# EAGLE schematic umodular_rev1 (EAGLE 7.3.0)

## Sheet 1 of 8: vco1
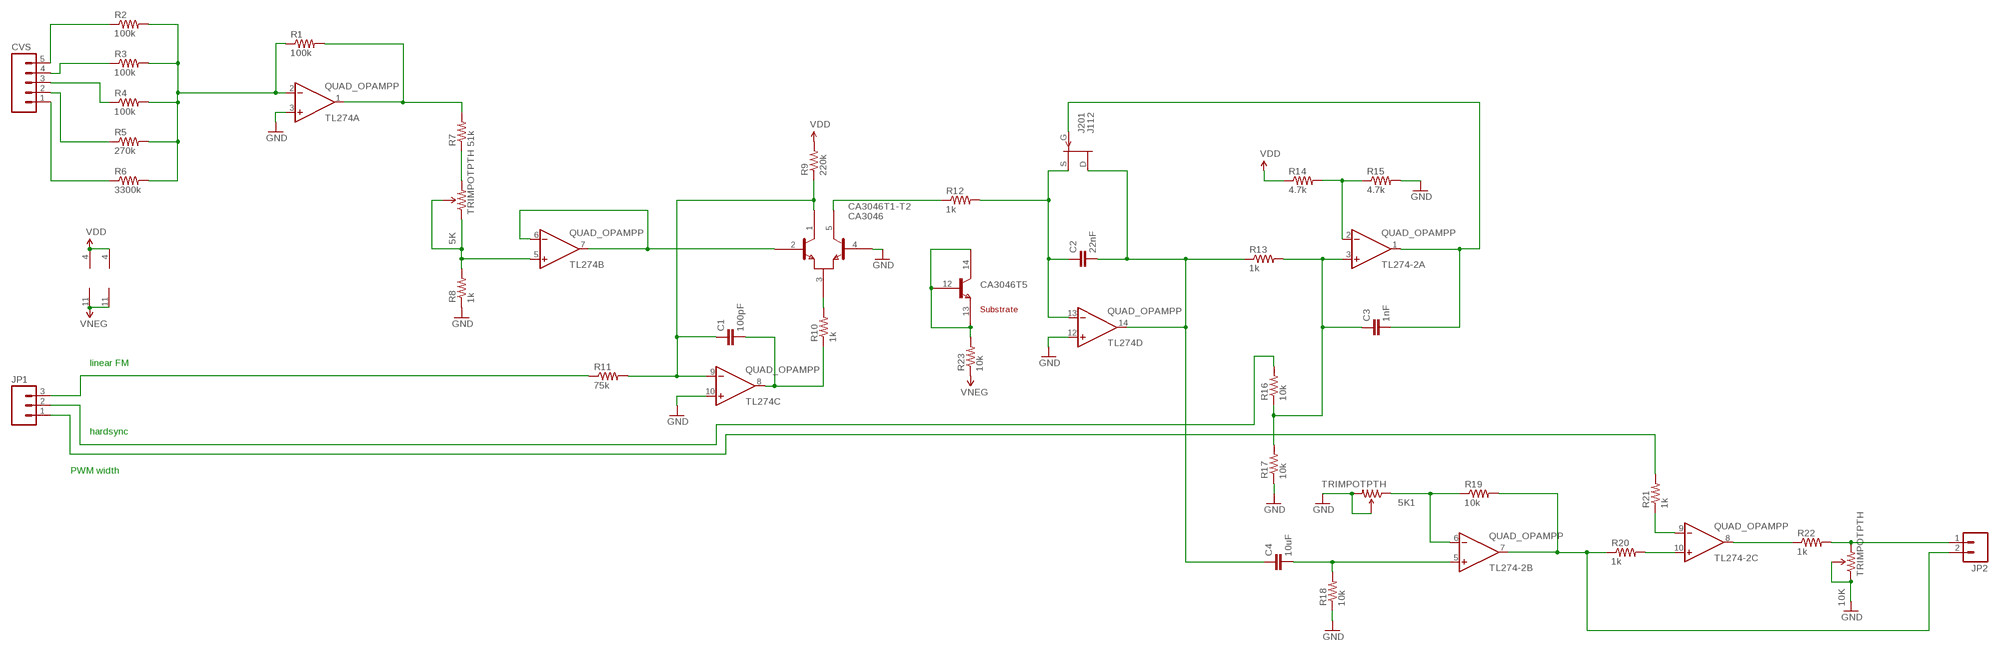
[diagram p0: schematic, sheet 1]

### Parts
5K  TRIMPOTPTH  [TRIM_POT_PTH]
5K1  TRIMPOTPTH  [TRIM_POT_PTH]
10K  TRIMPOTPTH  [TRIM_POT_PTH]
C1  100pF  CAPPTH  [CAP-PTH-SMALL]
C2  22nF  CAPPTH1  [CAP-PTH-5MM]
C3  1nF  CAPPTH  [CAP-PTH-SMALL]
C4  10uF  CAPPTH  [CAP-PTH-SMALL]
CA3046  CA3046  [DIL14]
CVS  M05LOCK_LONGPADS  [1X05_LOCK_LONGPADS]
J112  J201  [TO92]
JP1  M03LOCK_LONGPADS  [1X03_LOCK_LONGPADS]
JP2  M02LOCK_LONGPADS  [1X02_LOCK_LONGPADS]
R1  100k  RESISTORPTH-1/4W  [AXIAL-0.4]
R2  100k  RESISTORPTH-1/4W  [AXIAL-0.4]
R3  100k  RESISTORPTH-1/4W  [AXIAL-0.4]
R4  100k  RESISTORPTH-1/4W  [AXIAL-0.4]
R5  270k  RESISTORPTH-1/4W  [AXIAL-0.4]
R6  3300k  RESISTORPTH-1/4W  [AXIAL-0.4]
R7  51k  RESISTORPTH-1/4W  [AXIAL-0.4]
R8  1k  RESISTORPTH-1/4W  [AXIAL-0.4]
R9  220k  RESISTORPTH-1/4W  [AXIAL-0.4]
R10  1k  RESISTORPTH-1/4W  [AXIAL-0.4]
R11  75k  RESISTORPTH-1/4W  [AXIAL-0.4]
R12  1k  RESISTORPTH-1/4W  [AXIAL-0.4]
R13  1k  RESISTORPTH-1/4W  [AXIAL-0.4]
R14  4.7k  RESISTORPTH-1/4W  [AXIAL-0.4]
R15  4.7k  RESISTORPTH-1/4W  [AXIAL-0.4]
R16  10k  RESISTORPTH-1/4W  [AXIAL-0.4]
R17  10k  RESISTORPTH-1/4W  [AXIAL-0.4]
R18  10k  RESISTORPTH-1/4W  [AXIAL-0.4]
R19  10k  RESISTORPTH-1/4W  [AXIAL-0.4]
R20  1k  RESISTORPTH-1/4W  [AXIAL-0.4]
R21  1k  RESISTORPTH-1/4W  [AXIAL-0.4]
R22  1k  RESISTORPTH-1/4W  [AXIAL-0.4]
R23  10k  RESISTORPTH-1/4W  [AXIAL-0.4]
TL274  QUAD_OPAMPP  [DIL14]
TL274-2  QUAD_OPAMPP  [DIL14]

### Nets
GND: 5K1.2(WIPER) 5K1.3(CW) 10K.1(CCW) 10K.2(WIPER) CA3046.4(T1-T2:B2) R8.P$1 R15.P$2 R17.P$1 R18.P$1 TL274.3(A:+IN) TL274.10(C:+IN) TL274.12(D:+IN) ; also sheet 2,3,4,5,6,7,8
N$1: R1.P$1 R2.P$2 R3.P$2 R4.P$2 R5.P$2 R6.P$2 TL274.2(A:-IN)
N$2: R1.P$2 R7.P$2 TL274.1(A:OUT)
N$3: CVS.5 R2.P$1
N$4: CVS.4 R3.P$1
N$5: CVS.3 R4.P$1
N$6: CVS.2 R5.P$1
N$7: CVS.1 R6.P$1
N$8: 5K.3(CW) R7.P$1
N$9: 5K.1(CCW) 5K.2(WIPER) R8.P$2 TL274.5(B:+IN)
N$10: CA3046.2(T1-T2:B1) TL274.6(B:-IN) TL274.7(B:OUT)
N$11: JP1.3 R11.P$1
N$12: C1.2 R10.P$1 TL274.8(C:OUT)
N$13: CA3046.5(T1-T2:C2) R12.P$1
N$14: C1.1 CA3046.1(T1-T2:C1) R9.P$1 R11.P$2 TL274.9(C:-IN)
N$15: CA3046.3(T1-T2:E) R10.P$2
N$16: C2.1 J112.2(S) R12.P$2 TL274.13(D:-IN)
N$17: C2.2 C4.1 J112.3(D) R13.P$1 TL274.14(D:OUT)
N$18: R20.P$2 TL274-2.10(C:+IN)
N$19: C3.2 J112.1(G) TL274-2.1(A:OUT)
N$20: R21.P$1 TL274-2.9(C:-IN)
N$21: R14.P$2 R15.P$1 TL274-2.2(A:-IN)
N$22: JP1.1 R21.P$2
N$23: C3.1 R13.P$2 R16.P$1 R17.P$2 TL274-2.3(A:+IN)
N$24: JP1.2 R16.P$2
N$25: C4.2 R18.P$2 TL274-2.5(B:+IN)
N$26: 5K1.1(CCW) R19.P$1 TL274-2.6(B:-IN)
N$27: JP2.2 R19.P$2 R20.P$1 TL274-2.7(B:OUT)
N$28: R22.P$1 TL274-2.8(C:OUT)
N$29: 10K.3(CW) JP2.1 R22.P$2
N$31: CA3046.12(T5:B) CA3046.13(T5:E) CA3046.14(T5:C) R23.P$2
VDD: R9.P$2 R14.P$1 TL274-2.4(P:V+) TL274.4(P:V+) ; also sheet 2,3,4,5,6,7,8
VNEG: R23.P$1 TL274-2.11(P:V-) TL274.11(P:V-) ; also sheet 2,3,4,5,6,7,8
Unconnected: CA3046.6(T3:B) CA3046.7(T3:E) CA3046.8(T3:C) CA3046.9(T4:B) CA3046.10(T4:E) CA3046.11(T4:C) TL274-2.12(D:+IN) TL274-2.13(D:-IN) TL274-2.14(D:OUT)

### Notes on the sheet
- linear FM
- hardsync
- PWM width

## Sheet 2 of 8: vco2
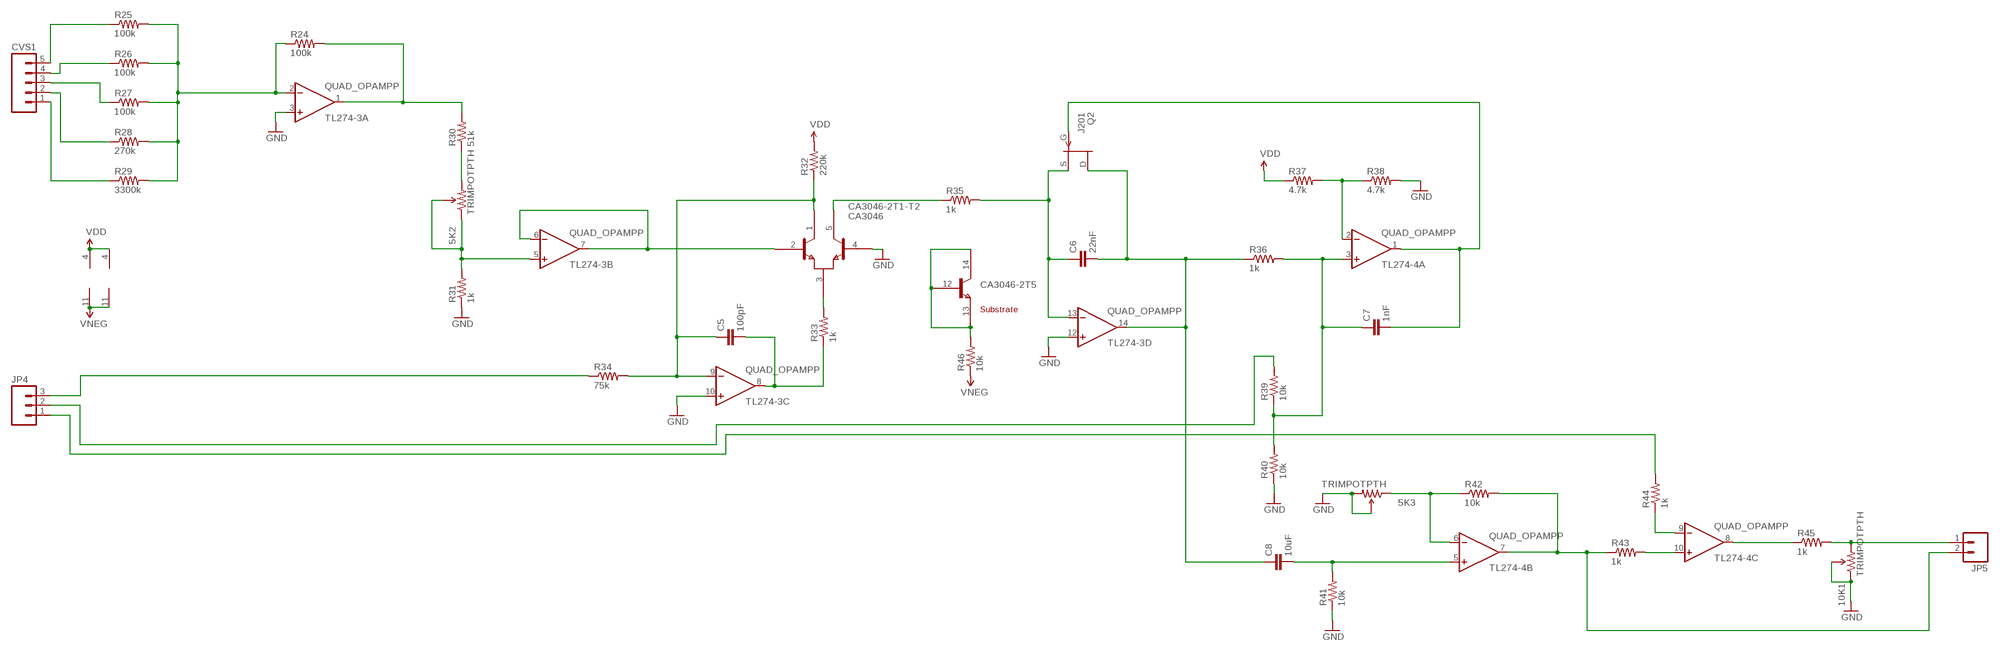
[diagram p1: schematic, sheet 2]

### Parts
5K2  TRIMPOTPTH  [TRIM_POT_PTH]
5K3  TRIMPOTPTH  [TRIM_POT_PTH]
10K1  TRIMPOTPTH  [TRIM_POT_PTH]
C5  100pF  CAPPTH  [CAP-PTH-SMALL]
C6  22nF  CAPPTH1  [CAP-PTH-5MM]
C7  1nF  CAPPTH  [CAP-PTH-SMALL]
C8  10uF  CAPPTH  [CAP-PTH-SMALL]
CA3046-2  CA3046  [DIL14]
CVS1  M05LOCK_LONGPADS  [1X05_LOCK_LONGPADS]
JP4  M03LOCK_LONGPADS  [1X03_LOCK_LONGPADS]
JP5  M02LOCK_LONGPADS  [1X02_LOCK_LONGPADS]
Q2  J201  [TO92]
R24  100k  RESISTORPTH-1/4W  [AXIAL-0.4]
R25  100k  RESISTORPTH-1/4W  [AXIAL-0.4]
R26  100k  RESISTORPTH-1/4W  [AXIAL-0.4]
R27  100k  RESISTORPTH-1/4W  [AXIAL-0.4]
R28  270k  RESISTORPTH-1/4W  [AXIAL-0.4]
R29  3300k  RESISTORPTH-1/4W  [AXIAL-0.4]
R30  51k  RESISTORPTH-1/4W  [AXIAL-0.4]
R31  1k  RESISTORPTH-1/4W  [AXIAL-0.4]
R32  220k  RESISTORPTH-1/4W  [AXIAL-0.4]
R33  1k  RESISTORPTH-1/4W  [AXIAL-0.4]
R34  75k  RESISTORPTH-1/4W  [AXIAL-0.4]
R35  1k  RESISTORPTH-1/4W  [AXIAL-0.4]
R36  1k  RESISTORPTH-1/4W  [AXIAL-0.4]
R37  4.7k  RESISTORPTH-1/4W  [AXIAL-0.4]
R38  4.7k  RESISTORPTH-1/4W  [AXIAL-0.4]
R39  10k  RESISTORPTH-1/4W  [AXIAL-0.4]
R40  10k  RESISTORPTH-1/4W  [AXIAL-0.4]
R41  10k  RESISTORPTH-1/4W  [AXIAL-0.4]
R42  10k  RESISTORPTH-1/4W  [AXIAL-0.4]
R43  1k  RESISTORPTH-1/4W  [AXIAL-0.4]
R44  1k  RESISTORPTH-1/4W  [AXIAL-0.4]
R45  1k  RESISTORPTH-1/4W  [AXIAL-0.4]
R46  10k  RESISTORPTH-1/4W  [AXIAL-0.4]
TL274-3  QUAD_OPAMPP  [DIL14]
TL274-4  QUAD_OPAMPP  [DIL14]

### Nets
GND: 5K3.2(WIPER) 5K3.3(CW) 10K1.1(CCW) 10K1.2(WIPER) CA3046-2.4(T1-T2:B2) R31.P$1 R38.P$2 R40.P$1 R41.P$1 TL274-3.3(A:+IN) TL274-3.10(C:+IN) TL274-3.12(D:+IN) ; also sheet 1,3,4,5,6,7,8
N$30: R24.P$1 R25.P$2 R26.P$2 R27.P$2 R28.P$2 R29.P$2 TL274-3.2(A:-IN)
N$32: R24.P$2 R30.P$2 TL274-3.1(A:OUT)
N$33: CVS1.5 R25.P$1
N$34: CVS1.4 R26.P$1
N$35: CVS1.3 R27.P$1
N$36: CVS1.2 R28.P$1
N$37: CVS1.1 R29.P$1
N$38: 5K2.3(CW) R30.P$1
N$39: 5K2.1(CCW) 5K2.2(WIPER) R31.P$2 TL274-3.5(B:+IN)
N$40: CA3046-2.2(T1-T2:B1) TL274-3.6(B:-IN) TL274-3.7(B:OUT)
N$41: C5.2 R33.P$1 TL274-3.8(C:OUT)
N$42: C5.1 CA3046-2.1(T1-T2:C1) R32.P$1 R34.P$2 TL274-3.9(C:-IN)
N$43: CA3046-2.3(T1-T2:E) R33.P$2
N$44: JP4.3 R34.P$1
N$45: CA3046-2.5(T1-T2:C2) R35.P$1
N$46: C6.1 Q2.2(S) R35.P$2 TL274-3.13(D:-IN)
N$47: C6.2 C8.1 Q2.3(D) R36.P$1 TL274-3.14(D:OUT)
N$48: C7.2 Q2.1(G) TL274-4.1(A:OUT)
N$49: R37.P$2 R38.P$1 TL274-4.2(A:-IN)
N$50: C7.1 R36.P$2 R39.P$1 R40.P$2 TL274-4.3(A:+IN)
N$51: JP4.2 R39.P$2
N$52: C8.2 R41.P$2 TL274-4.5(B:+IN)
N$53: 5K3.1(CCW) R42.P$1 TL274-4.6(B:-IN)
N$54: JP5.2 R42.P$2 R43.P$1 TL274-4.7(B:OUT)
N$55: R43.P$2 TL274-4.10(C:+IN)
N$56: R44.P$1 TL274-4.9(C:-IN)
N$57: JP4.1 R44.P$2
N$58: R45.P$1 TL274-4.8(C:OUT)
N$59: 10K1.3(CW) JP5.1 R45.P$2
N$60: CA3046-2.12(T5:B) CA3046-2.13(T5:E) CA3046-2.14(T5:C) R46.P$2
VDD: R32.P$2 R37.P$1 TL274-3.4(P:V+) TL274-4.4(P:V+) ; also sheet 1,3,4,5,6,7,8
VNEG: R46.P$1 TL274-3.11(P:V-) TL274-4.11(P:V-) ; also sheet 1,3,4,5,6,7,8
Unconnected: CA3046-2.6(T3:B) CA3046-2.7(T3:E) CA3046-2.8(T3:C) CA3046-2.9(T4:B) CA3046-2.10(T4:E) CA3046-2.11(T4:C) TL274-4.12(D:+IN) TL274-4.13(D:-IN) TL274-4.14(D:OUT)

## Sheet 3 of 8: pwr
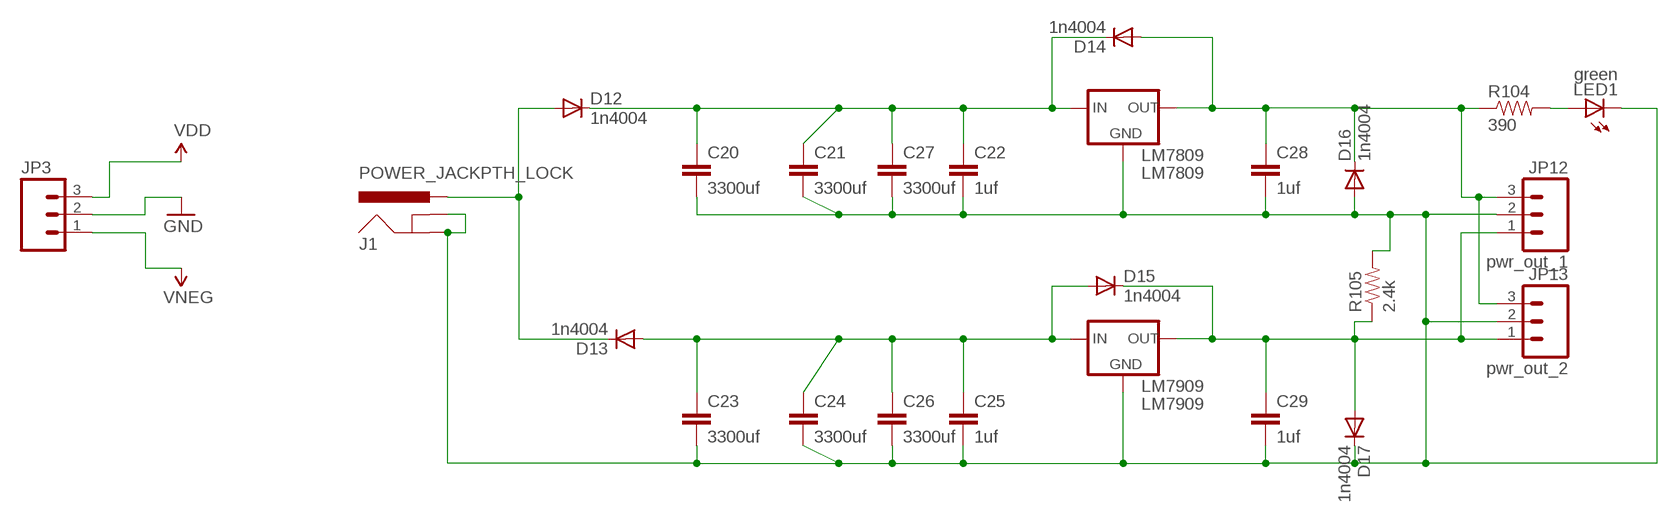
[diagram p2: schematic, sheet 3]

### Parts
C20  3300uf  CAPPTH3  [CAP-PTH-LARGE]
C21  3300uf  CAPPTH3  [CAP-PTH-LARGE]
C22  1uf  CAPPTH1  [CAP-PTH-5MM]
C23  3300uf  CAPPTH3  [CAP-PTH-LARGE]
C24  3300uf  CAPPTH3  [CAP-PTH-LARGE]
C25  1uf  CAPPTH1  [CAP-PTH-5MM]
C26  3300uf  CAPPTH3  [CAP-PTH-LARGE]
C27  3300uf  CAPPTH3  [CAP-PTH-LARGE]
C28  1uf  CAPPTH1  [CAP-PTH-5MM]
C29  1uf  CAPPTH1  [CAP-PTH-5MM]
D12  1n4004  DIODEPTH  [DIODE-1N4001]
D13  1n4004  DIODEPTH  [DIODE-1N4001]
D14  1n4004  DIODEPTH  [DIODE-1N4001]
D15  1n4004  DIODEPTH  [DIODE-1N4001]
D16  1n4004  DIODEPTH  [DIODE-1N4001]
D17  1n4004  DIODEPTH  [DIODE-1N4001]
J1  POWER_JACKPTH_LOCK  [POWER_JACK_PTH_LOCK]
JP3  M03LOCK_LONGPADS  [1X03_LOCK_LONGPADS]
JP12  pwr_out_1  M03LOCK_LONGPADS  [1X03_LOCK_LONGPADS]
JP13  pwr_out_2  M03LOCK_LONGPADS  [1X03_LOCK_LONGPADS]
LED1  green  LED3MM  [LED3MM]
LM7809  LM7809  V_REG_78XX-TO-220  [TO-220-ALT]
LM7909  LM7909  V_REG_78XX-TO-220  [TO-220-ALT]
R104  390  RESISTORPTH-1/4W  [AXIAL-0.4]
R105  2.4k  RESISTORPTH-1/4W  [AXIAL-0.4]

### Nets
GND: JP3.2 ; also sheet 1,2,4,5,6,7,8
N$150: D12.A D13.C J1.PWR
N$151: C20.1 C21.1 C22.1 C27.1 D12.C D14.C LM7809.IN
N$152: C20.2 C21.2 C22.2 C23.2 C24.2 C25.2 C26.2 C27.2 C28.2 C29.2 D16.A D17.C J1.GND J1.GNDBREAK JP12.2 JP13.2 LED1.K(C) LM7809.GND LM7909.GND R105.P$2
N$153: C23.1 C24.1 C25.1 C26.1 D13.A D15.A LM7909.IN
N$155: C28.1 D14.A D16.C JP12.3 JP13.3 LM7809.OUT R104.P$1
N$156: C29.1 D15.C D17.A JP12.1 JP13.1 LM7909.OUT R105.P$1
N$159: LED1.A R104.P$2
VDD: JP3.3 ; also sheet 1,2,4,5,6,7,8
VNEG: JP3.1 ; also sheet 1,2,4,5,6,7,8

## Sheet 4 of 8: vcf
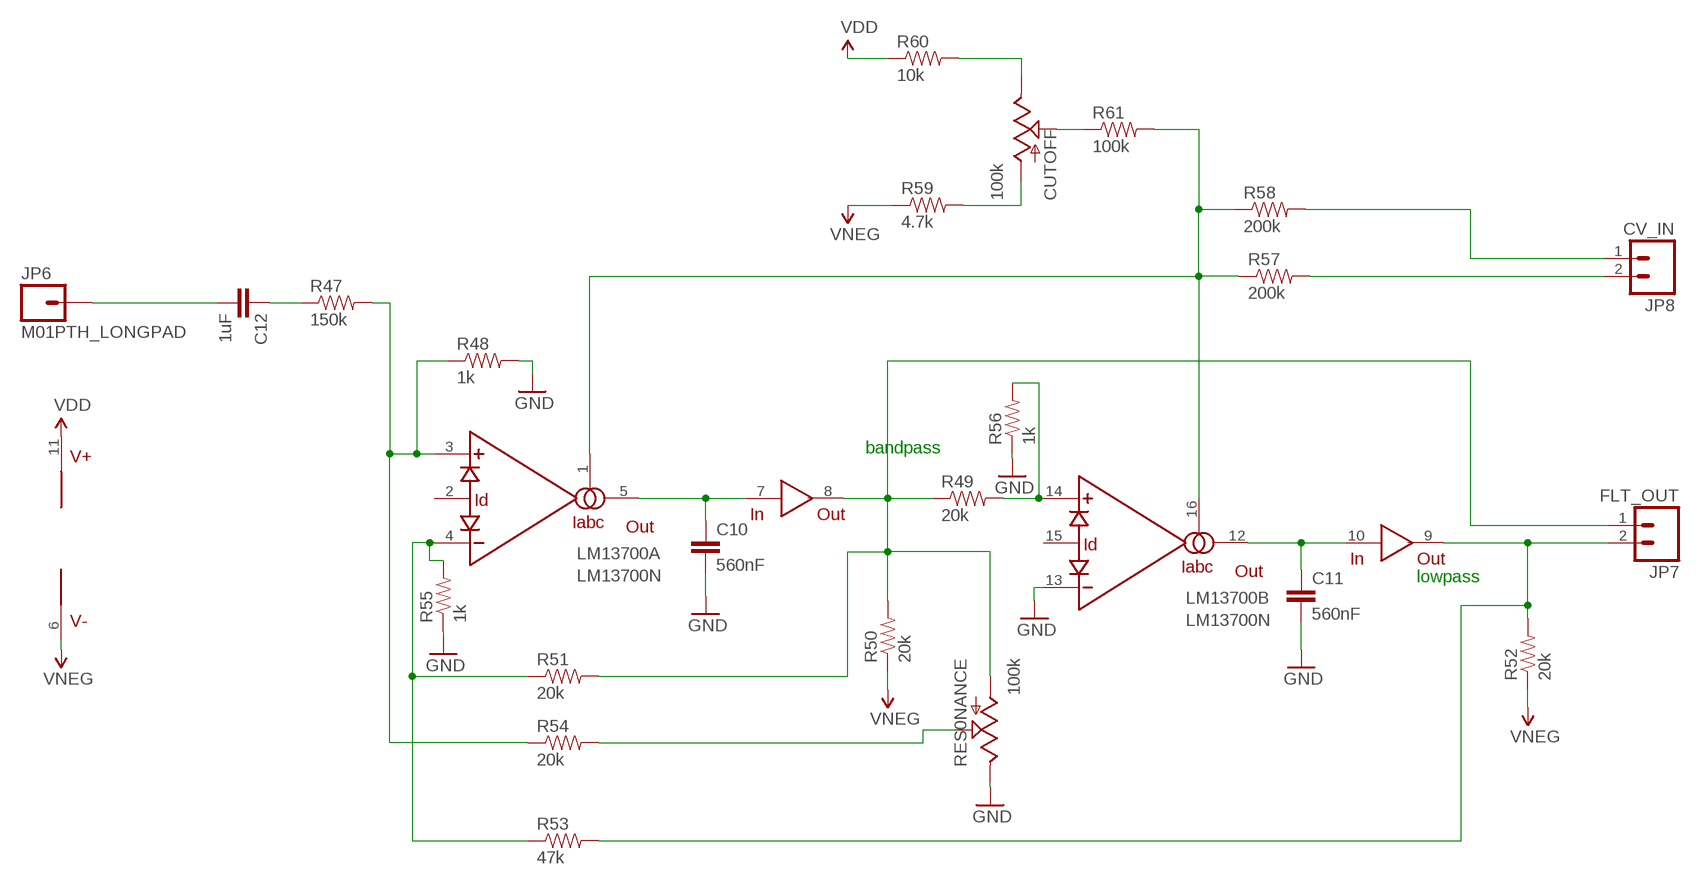
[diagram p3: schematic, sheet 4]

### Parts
C10  560nF  CAPPTH  [CAP-PTH-SMALL]
C11  560nF  CAPPTH  [CAP-PTH-SMALL]
C12  1uF  CAPPTH1  [CAP-PTH-5MM]
CUTOFF  100k  POTALPS-KIT  [ALPS_POT_KIT]
JP6  M01PTH_LONGPAD  [1X01_LONGPAD]
JP7  FLT_OUT  M02LOCK_LONGPADS  [1X02_LOCK_LONGPADS]
JP8  CV_IN  M02LOCK_LONGPADS  [1X02_LOCK_LONGPADS]
LM13700  LM13700N  [DIL16]
R47  150k  RESISTORPTH-1/4W  [AXIAL-0.4]
R48  1k  RESISTORPTH-1/4W  [AXIAL-0.4]
R49  20k  RESISTORPTH-1/4W  [AXIAL-0.4]
R50  20k  RESISTORPTH-1/4W  [AXIAL-0.4]
R51  20k  RESISTORPTH-1/4W  [AXIAL-0.4]
R52  20k  RESISTORPTH-1/4W  [AXIAL-0.4]
R53  47k  RESISTORPTH-1/4W  [AXIAL-0.4]
R54  20k  RESISTORPTH-1/4W  [AXIAL-0.4]
R55  1k  RESISTORPTH-1/4W  [AXIAL-0.4]
R56  1k  RESISTORPTH-1/4W  [AXIAL-0.4]
R57  200k  RESISTORPTH-1/4W  [AXIAL-0.4]
R58  200k  RESISTORPTH-1/4W  [AXIAL-0.4]
R59  4.7k  RESISTORPTH-1/4W  [AXIAL-0.4]
R60  10k  RESISTORPTH-1/4W  [AXIAL-0.4]
R61  100k  RESISTORPTH-1/4W  [AXIAL-0.4]
RES0NANCE  100k  POTALPS-KIT  [ALPS_POT_KIT]

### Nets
GND: C10.2 C11.2 LM13700.13(B:-IN) R48.P$2 R55.P$1 R56.P$1 RES0NANCE.P$1(E) ; also sheet 1,2,3,5,6,7,8
N$61: C12.2 JP6.1
N$62: C12.1 R47.P$1
N$63: C10.1 LM13700.5(A:OUT) LM13700.7(IN)
N$64: LM13700.3(A:+IN) R47.P$2 R48.P$1 R54.P$1
N$65: JP7.1 LM13700.8(OUT) R49.P$1 R50.P$2 R51.P$2 RES0NANCE.P$3(A)
N$66: LM13700.14(B:+IN) R49.P$2 R56.P$2
N$67: LM13700.4(A:-IN) R51.P$1 R53.P$1 R55.P$2
N$68: JP7.2 LM13700.9(OUT) R52.P$2 R53.P$2
N$69: C11.1 LM13700.10(IN) LM13700.12(B:OUT)
N$70: LM13700.1(A:IABC) LM13700.16(B:IABC) R57.P$1 R58.P$1 R61.P$2
N$71: R54.P$2 RES0NANCE.P$2(S)
N$72: JP8.2 R57.P$2
N$73: JP8.1 R58.P$2
N$74: CUTOFF.P$1(E) R60.P$2
N$75: CUTOFF.P$3(A) R59.P$2
N$76: CUTOFF.P$2(S) R61.P$1
VDD: LM13700.11(V+) R60.P$1 ; also sheet 1,2,3,5,6,7,8
VNEG: LM13700.6(V-) R50.P$1 R52.P$1 R59.P$1 ; also sheet 1,2,3,5,6,7,8
Unconnected: LM13700.2(A:ID) LM13700.15(B:ID)

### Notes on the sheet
- bandpass
- lowpass

## Sheet 5 of 8: adsr1
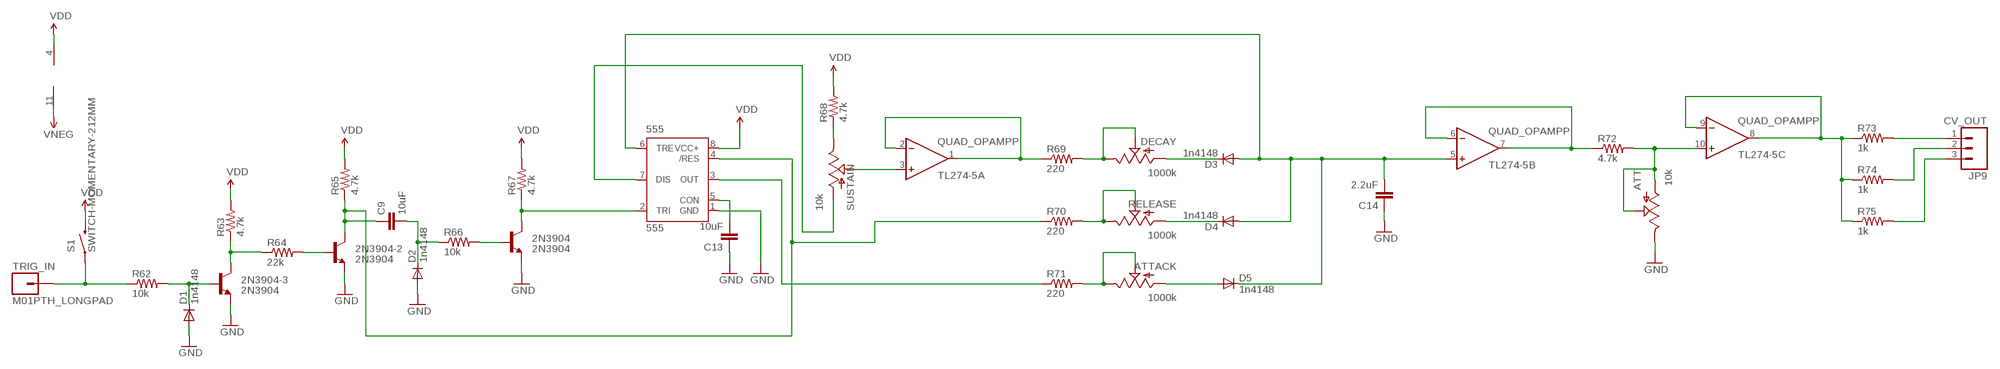
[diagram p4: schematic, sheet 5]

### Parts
2N3904  2N3904  TRANSISTOR_NPNTO-92-AMMO  [TO-92-AMMO]
2N3904-2  2N3904  TRANSISTOR_NPNTO-92-AMMO  [TO-92-AMMO]
2N3904-3  2N3904  TRANSISTOR_NPNTO-92-AMMO  [TO-92-AMMO]
555  555  NE555P  [DIL-08]
ATT  10k  POTALPS-KIT  [ALPS_POT_KIT]
ATTACK  1000k  POTALPS-KIT  [ALPS_POT_KIT]
C9  10uF  CAPPTH1  [CAP-PTH-5MM]
C13  10uF  CAPPTH1  [CAP-PTH-5MM]
C14  2.2uF  CAPPTH1  [CAP-PTH-5MM]
D1  1n4148  DIODE1N4148  [DIODE-1N4148]
D2  1n4148  DIODE1N4148  [DIODE-1N4148]
D3  1n4148  DIODE1N4148  [DIODE-1N4148]
D4  1n4148  DIODE1N4148  [DIODE-1N4148]
D5  1n4148  DIODE1N4148  [DIODE-1N4148]
DECAY  1000k  POTALPS-KIT  [ALPS_POT_KIT]
JP9  CV_OUT  M03LOCK_LONGPADS  [1X03_LOCK_LONGPADS]
R62  10k  RESISTORPTH-1/4W  [AXIAL-0.4]
R63  4.7k  RESISTORPTH-1/4W  [AXIAL-0.4]
R64  22k  RESISTORPTH-1/4W  [AXIAL-0.4]
R65  4.7k  RESISTORPTH-1/4W  [AXIAL-0.4]
R66  10k  RESISTORPTH-1/4W  [AXIAL-0.4]
R67  4.7k  RESISTORPTH-1/4W  [AXIAL-0.4]
R68  4.7k  RESISTORPTH-1/4W  [AXIAL-0.4]
R69  220  RESISTORPTH-1/4W  [AXIAL-0.4]
R70  220  RESISTORPTH-1/4W  [AXIAL-0.4]
R71  220  RESISTORPTH-1/4W  [AXIAL-0.4]
R72  4.7k  RESISTORPTH-1/4W  [AXIAL-0.4]
R73  1k  RESISTORPTH-1/4W  [AXIAL-0.4]
R74  1k  RESISTORPTH-1/4W  [AXIAL-0.4]
R75  1k  RESISTORPTH-1/4W  [AXIAL-0.4]
RELEASE  1000k  POTALPS-KIT  [ALPS_POT_KIT]
S1  SWITCH-MOMENTARY-212MM  [TACTILE-PTH-12MM]
SUSTAIN  10k  POTALPS-KIT  [ALPS_POT_KIT]
TL274-5  QUAD_OPAMPP  [DIL14]
TRIG_IN  M01PTH_LONGPAD  [1X01_LONGPAD]

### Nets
GND: 2N3904-2.1(E) 2N3904-3.1(E) 2N3904.1(E) 555.1(GND) ATT.P$1(E) C13.1 C14.1 D1.A D2.A ; also sheet 1,2,3,4,6,7,8
N$77: R62.P$1 S1.1 TRIG_IN.1
N$78: 2N3904-3.2(B) D1.C R62.P$2
N$79: 2N3904.3(C) 555.2(TRI) R67.P$1
N$80: 2N3904-2.3(C) 555.4(/RES) C9.1 R65.P$1 R70.P$1
N$81: 2N3904-3.3(C) R63.P$1 R64.P$1
N$82: 2N3904-2.2(B) R64.P$2
N$83: C9.2 D2.C R66.P$1
N$84: 2N3904.2(B) R66.P$2
N$85: SUSTAIN.P$2(S) TL274-5.3(A:+IN)
N$86: 555.5(CON) C13.2
N$87: 555.7(DIS) SUSTAIN.P$3(A)
N$88: R68.P$1 SUSTAIN.P$1(E)
N$89: R69.P$1 TL274-5.1(A:OUT) TL274-5.2(A:-IN)
N$90: DECAY.P$1(E) DECAY.P$2(S) R69.P$2
N$91: D3.C DECAY.P$3(A)
N$92: 555.6(TRE) C14.2 D3.A D4.A D5.C TL274-5.5(B:+IN)
N$93: 555.3(OUT) R71.P$1
N$94: ATTACK.P$1(E) ATTACK.P$2(S) R71.P$2
N$95: R70.P$2 RELEASE.P$1(E) RELEASE.P$2(S)
N$96: D4.C RELEASE.P$3(A)
N$97: ATTACK.P$3(A) D5.A
N$98: R72.P$1 TL274-5.6(B:-IN) TL274-5.7(B:OUT)
N$99: ATT.P$2(S) ATT.P$3(A) R72.P$2 TL274-5.10(C:+IN)
N$100: R73.P$1 R74.P$1 R75.P$1 TL274-5.8(C:OUT) TL274-5.9(C:-IN)
N$101: JP9.1 R73.P$2
N$102: JP9.2 R74.P$2
N$103: JP9.3 R75.P$2
VDD: 555.8(VCC+) R63.P$2 R65.P$2 R67.P$2 R68.P$2 S1.3 TL274-5.4(P:V+) ; also sheet 1,2,3,4,6,7,8
VNEG: TL274-5.11(P:V-) ; also sheet 1,2,3,4,6,7,8
Unconnected: TL274-5.12(D:+IN) TL274-5.13(D:-IN) TL274-5.14(D:OUT)

## Sheet 6 of 8: adsr2
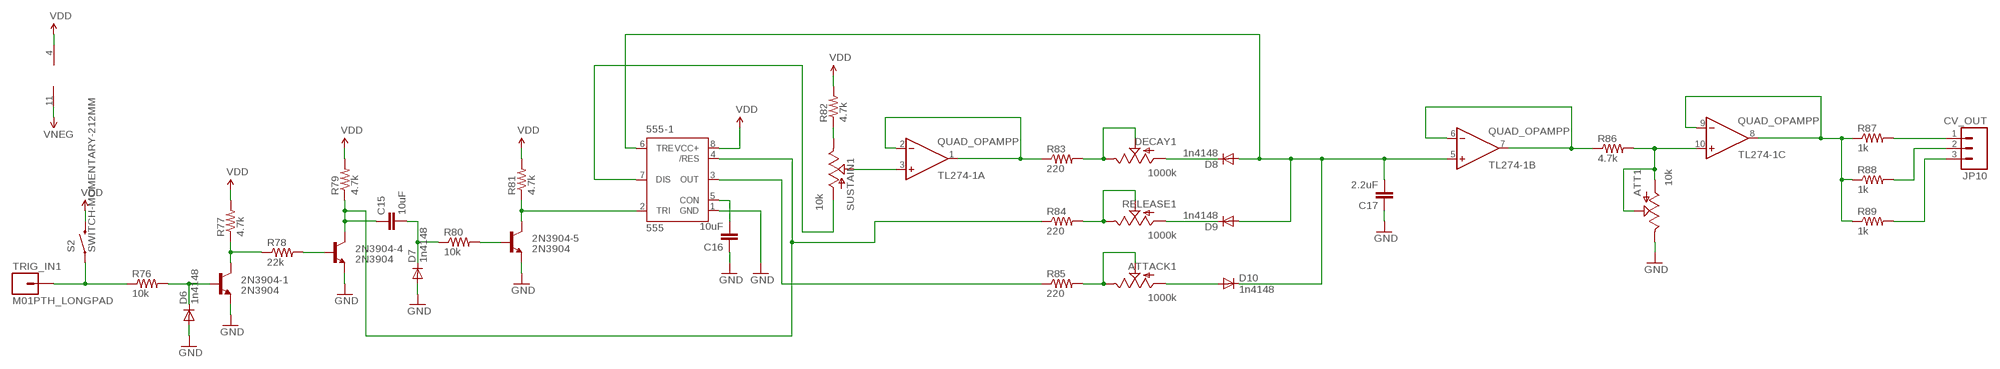
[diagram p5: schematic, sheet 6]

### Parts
2N3904-1  2N3904  TRANSISTOR_NPNTO-92-AMMO  [TO-92-AMMO]
2N3904-4  2N3904  TRANSISTOR_NPNTO-92-AMMO  [TO-92-AMMO]
2N3904-5  2N3904  TRANSISTOR_NPNTO-92-AMMO  [TO-92-AMMO]
555-1  555  NE555P  [DIL-08]
ATT1  10k  POTALPS-KIT  [ALPS_POT_KIT]
ATTACK1  1000k  POTALPS-KIT  [ALPS_POT_KIT]
C15  10uF  CAPPTH1  [CAP-PTH-5MM]
C16  10uF  CAPPTH1  [CAP-PTH-5MM]
C17  2.2uF  CAPPTH1  [CAP-PTH-5MM]
D6  1n4148  DIODE1N4148  [DIODE-1N4148]
D7  1n4148  DIODE1N4148  [DIODE-1N4148]
D8  1n4148  DIODE1N4148  [DIODE-1N4148]
D9  1n4148  DIODE1N4148  [DIODE-1N4148]
D10  1n4148  DIODE1N4148  [DIODE-1N4148]
DECAY1  1000k  POTALPS-KIT  [ALPS_POT_KIT]
JP10  CV_OUT  M03LOCK_LONGPADS  [1X03_LOCK_LONGPADS]
R76  10k  RESISTORPTH-1/4W  [AXIAL-0.4]
R77  4.7k  RESISTORPTH-1/4W  [AXIAL-0.4]
R78  22k  RESISTORPTH-1/4W  [AXIAL-0.4]
R79  4.7k  RESISTORPTH-1/4W  [AXIAL-0.4]
R80  10k  RESISTORPTH-1/4W  [AXIAL-0.4]
R81  4.7k  RESISTORPTH-1/4W  [AXIAL-0.4]
R82  4.7k  RESISTORPTH-1/4W  [AXIAL-0.4]
R83  220  RESISTORPTH-1/4W  [AXIAL-0.4]
R84  220  RESISTORPTH-1/4W  [AXIAL-0.4]
R85  220  RESISTORPTH-1/4W  [AXIAL-0.4]
R86  4.7k  RESISTORPTH-1/4W  [AXIAL-0.4]
R87  1k  RESISTORPTH-1/4W  [AXIAL-0.4]
R88  1k  RESISTORPTH-1/4W  [AXIAL-0.4]
R89  1k  RESISTORPTH-1/4W  [AXIAL-0.4]
RELEASE1  1000k  POTALPS-KIT  [ALPS_POT_KIT]
S2  SWITCH-MOMENTARY-212MM  [TACTILE-PTH-12MM]
SUSTAIN1  10k  POTALPS-KIT  [ALPS_POT_KIT]
TL274-1  QUAD_OPAMPP  [DIL14]
TRIG_IN1  M01PTH_LONGPAD  [1X01_LONGPAD]

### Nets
GND: 2N3904-1.1(E) 2N3904-4.1(E) 2N3904-5.1(E) 555-1.1(GND) ATT1.P$1(E) C16.1 C17.1 D6.A D7.A ; also sheet 1,2,3,4,5,7,8
N$104: R76.P$1 S2.1 TRIG_IN1.1
N$105: 2N3904-1.2(B) D6.C R76.P$2
N$106: 2N3904-5.3(C) 555-1.2(TRI) R81.P$1
N$107: 2N3904-4.3(C) 555-1.4(/RES) C15.1 R79.P$1 R84.P$1
N$108: 2N3904-1.3(C) R77.P$1 R78.P$1
N$109: 2N3904-4.2(B) R78.P$2
N$110: C15.2 D7.C R80.P$1
N$111: 2N3904-5.2(B) R80.P$2
N$112: 555-1.5(CON) C16.2
N$113: 555-1.7(DIS) SUSTAIN1.P$3(A)
N$114: R82.P$1 SUSTAIN1.P$1(E)
N$115: SUSTAIN1.P$2(S) TL274-1.3(A:+IN)
N$116: R83.P$1 TL274-1.1(A:OUT) TL274-1.2(A:-IN)
N$117: DECAY1.P$1(E) DECAY1.P$2(S) R83.P$2
N$118: D8.C DECAY1.P$3(A)
N$119: 555-1.6(TRE) C17.2 D8.A D9.A D10.C TL274-1.5(B:+IN)
N$120: R84.P$2 RELEASE1.P$1(E) RELEASE1.P$2(S)
N$121: D9.C RELEASE1.P$3(A)
N$122: 555-1.3(OUT) R85.P$1
N$123: ATTACK1.P$1(E) ATTACK1.P$2(S) R85.P$2
N$124: ATTACK1.P$3(A) D10.A
N$125: R86.P$1 TL274-1.6(B:-IN) TL274-1.7(B:OUT)
N$126: ATT1.P$2(S) ATT1.P$3(A) R86.P$2 TL274-1.10(C:+IN)
N$127: R87.P$1 R88.P$1 R89.P$1 TL274-1.8(C:OUT) TL274-1.9(C:-IN)
N$128: JP10.1 R87.P$2
N$129: JP10.2 R88.P$2
N$130: JP10.3 R89.P$2
VDD: 555-1.8(VCC+) R77.P$2 R79.P$2 R81.P$2 R82.P$2 S2.3 TL274-1.4(P:V+) ; also sheet 1,2,3,4,5,7,8
VNEG: TL274-1.11(P:V-) ; also sheet 1,2,3,4,5,7,8
Unconnected: TL274-1.12(D:+IN) TL274-1.13(D:-IN) TL274-1.14(D:OUT)

## Sheet 7 of 8: vca
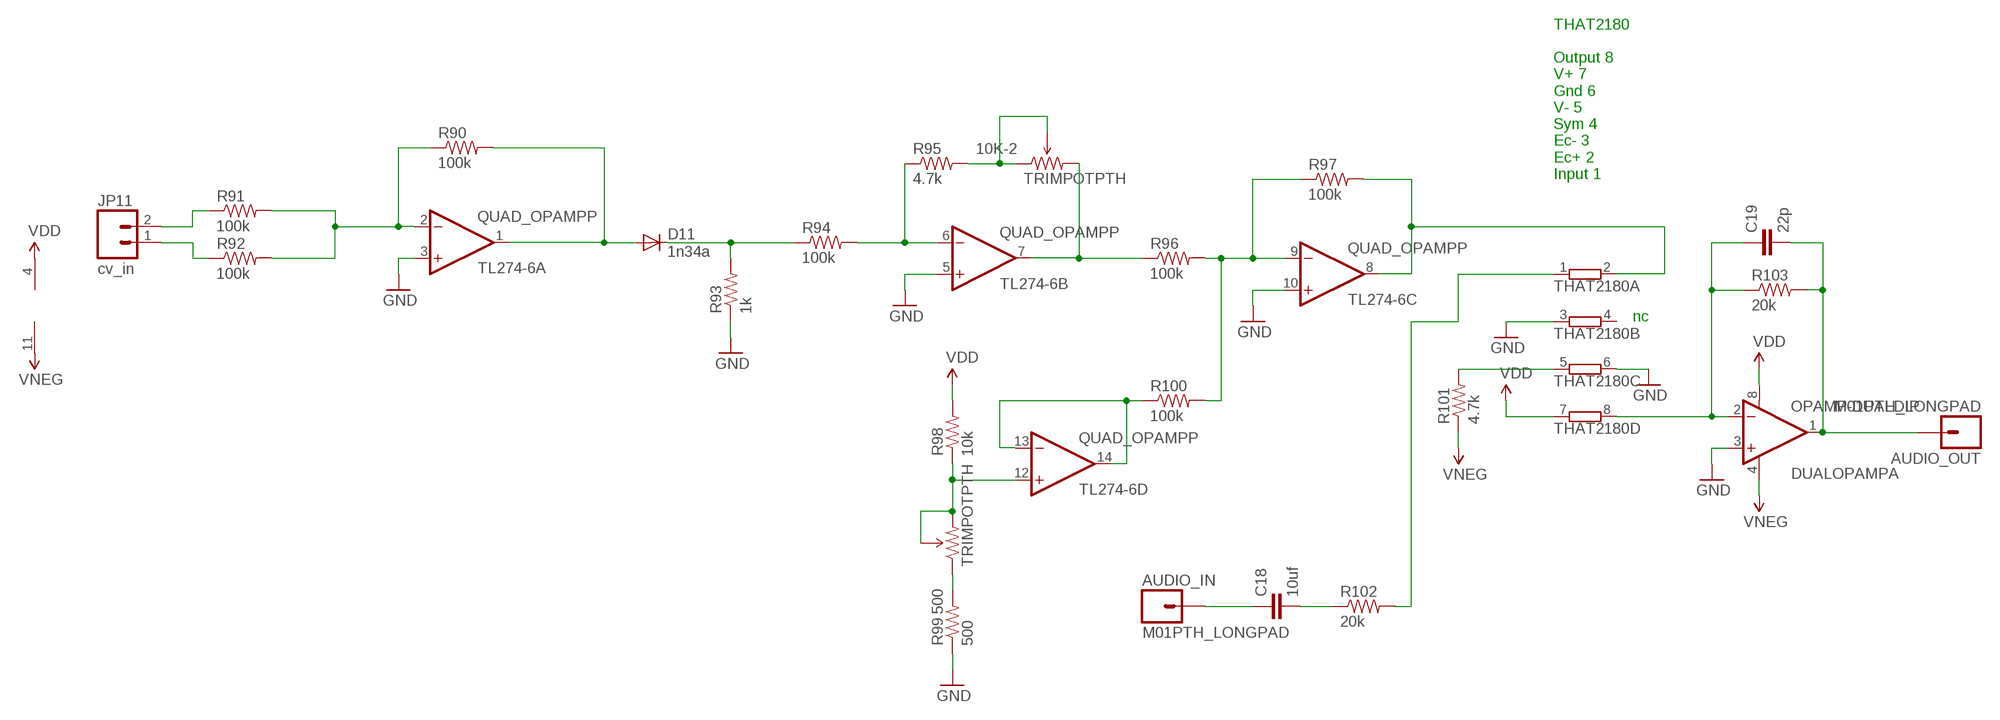
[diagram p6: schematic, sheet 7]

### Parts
10K-2  TRIMPOTPTH  [TRIM_POT_PTH]
500  TRIMPOTPTH  [TRIM_POT_PTH]
AUDIO_IN  M01PTH_LONGPAD  [1X01_LONGPAD]
AUDIO_OUT  M01PTH_LONGPAD  [1X01_LONGPAD]
C18  10uf  CAPPTH1  [CAP-PTH-5MM]
C19  22p  CAPPTH2  [CAP-PTH-SMALL2]
D11  1n34a  DIODE1N4148  [DIODE-1N4148]
DUALOPAMP  OPAMP-DUALDIP  [DIP08]
JP11  cv_in  M02LOCK_LONGPADS  [1X02_LOCK_LONGPADS]
R90  100k  RESISTORPTH-1/4W  [AXIAL-0.4]
R91  100k  RESISTORPTH-1/4W  [AXIAL-0.4]
R92  100k  RESISTORPTH-1/4W  [AXIAL-0.4]
R93  1k  RESISTORPTH-1/4W  [AXIAL-0.4]
R94  100k  RESISTORPTH-1/4W  [AXIAL-0.4]
R95  4.7k  RESISTORPTH-1/4W  [AXIAL-0.4]
R96  100k  RESISTORPTH-1/4W  [AXIAL-0.4]
R97  100k  RESISTORPTH-1/4W  [AXIAL-0.4]
R98  10k  RESISTORPTH-1/4W  [AXIAL-0.4]
R99  500  RESISTORPTH-1/4W  [AXIAL-0.4]
R100  100k  RESISTORPTH-1/4W  [AXIAL-0.4]
R101  4.7k  RESISTORPTH-1/4W  [AXIAL-0.4]
R102  20k  RESISTORPTH-1/4W  [AXIAL-0.4]
R103  20k  RESISTORPTH-1/4W  [AXIAL-0.4]
THAT2180  E4R  [SIL8]
TL274-6  QUAD_OPAMPP  [DIL14]

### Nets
GND: DUALOPAMP.3(A:+IN) R93.P$1 R99.P$1 THAT2180.3 THAT2180.6 TL274-6.3(A:+IN) TL274-6.5(B:+IN) TL274-6.10(C:+IN) ; also sheet 1,2,3,4,5,6,8
N$131: R90.P$1 R91.P$2 R92.P$2 TL274-6.2(A:-IN)
N$132: D11.A R90.P$2 TL274-6.1(A:OUT)
N$133: JP11.2 R91.P$1
N$134: JP11.1 R92.P$1
N$135: R94.P$2 R95.P$1 TL274-6.6(B:-IN)
N$136: 10K-2.1(CCW) 10K-2.2(WIPER) R95.P$2
N$137: D11.C R93.P$2 R94.P$1
N$138: 10K-2.3(CW) R96.P$1 TL274-6.7(B:OUT)
N$139: R96.P$2 R97.P$1 R100.P$2 TL274-6.9(C:-IN)
N$140: R97.P$2 THAT2180.2 TL274-6.8(C:OUT)
N$141: 500.2(WIPER) 500.3(CW) R98.P$1 TL274-6.12(D:+IN)
N$142: 500.1(CCW) R99.P$2
N$143: R100.P$1 TL274-6.13(D:-IN) TL274-6.14(D:OUT)
N$144: R101.P$2 THAT2180.5
N$145: AUDIO_IN.1 C18.1
N$146: C18.2 R102.P$1
N$147: R102.P$2 THAT2180.1
N$148: C19.1 DUALOPAMP.2(A:-IN) R103.P$1 THAT2180.8
N$149: AUDIO_OUT.1 C19.2 DUALOPAMP.1(A:OUT) R103.P$2
VDD: DUALOPAMP.8(A:V+) R98.P$2 THAT2180.7 TL274-6.4(P:V+) ; also sheet 1,2,3,4,5,6,8
VNEG: DUALOPAMP.4(A:V-) R101.P$1 TL274-6.11(P:V-) ; also sheet 1,2,3,4,5,6,8
Unconnected: DUALOPAMP.5(B:+IN) DUALOPAMP.6(B:-IN) DUALOPAMP.7(B:OUT) THAT2180.4

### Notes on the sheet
- THAT2180
  
  Output 8 
  V+ 7 
  Gnd 6 
  V- 5 
  Sym 4 
  Ec- 3 
  Ec+ 2 
  Input 1
- nc

## Sheet 8 of 8: mixer_cv
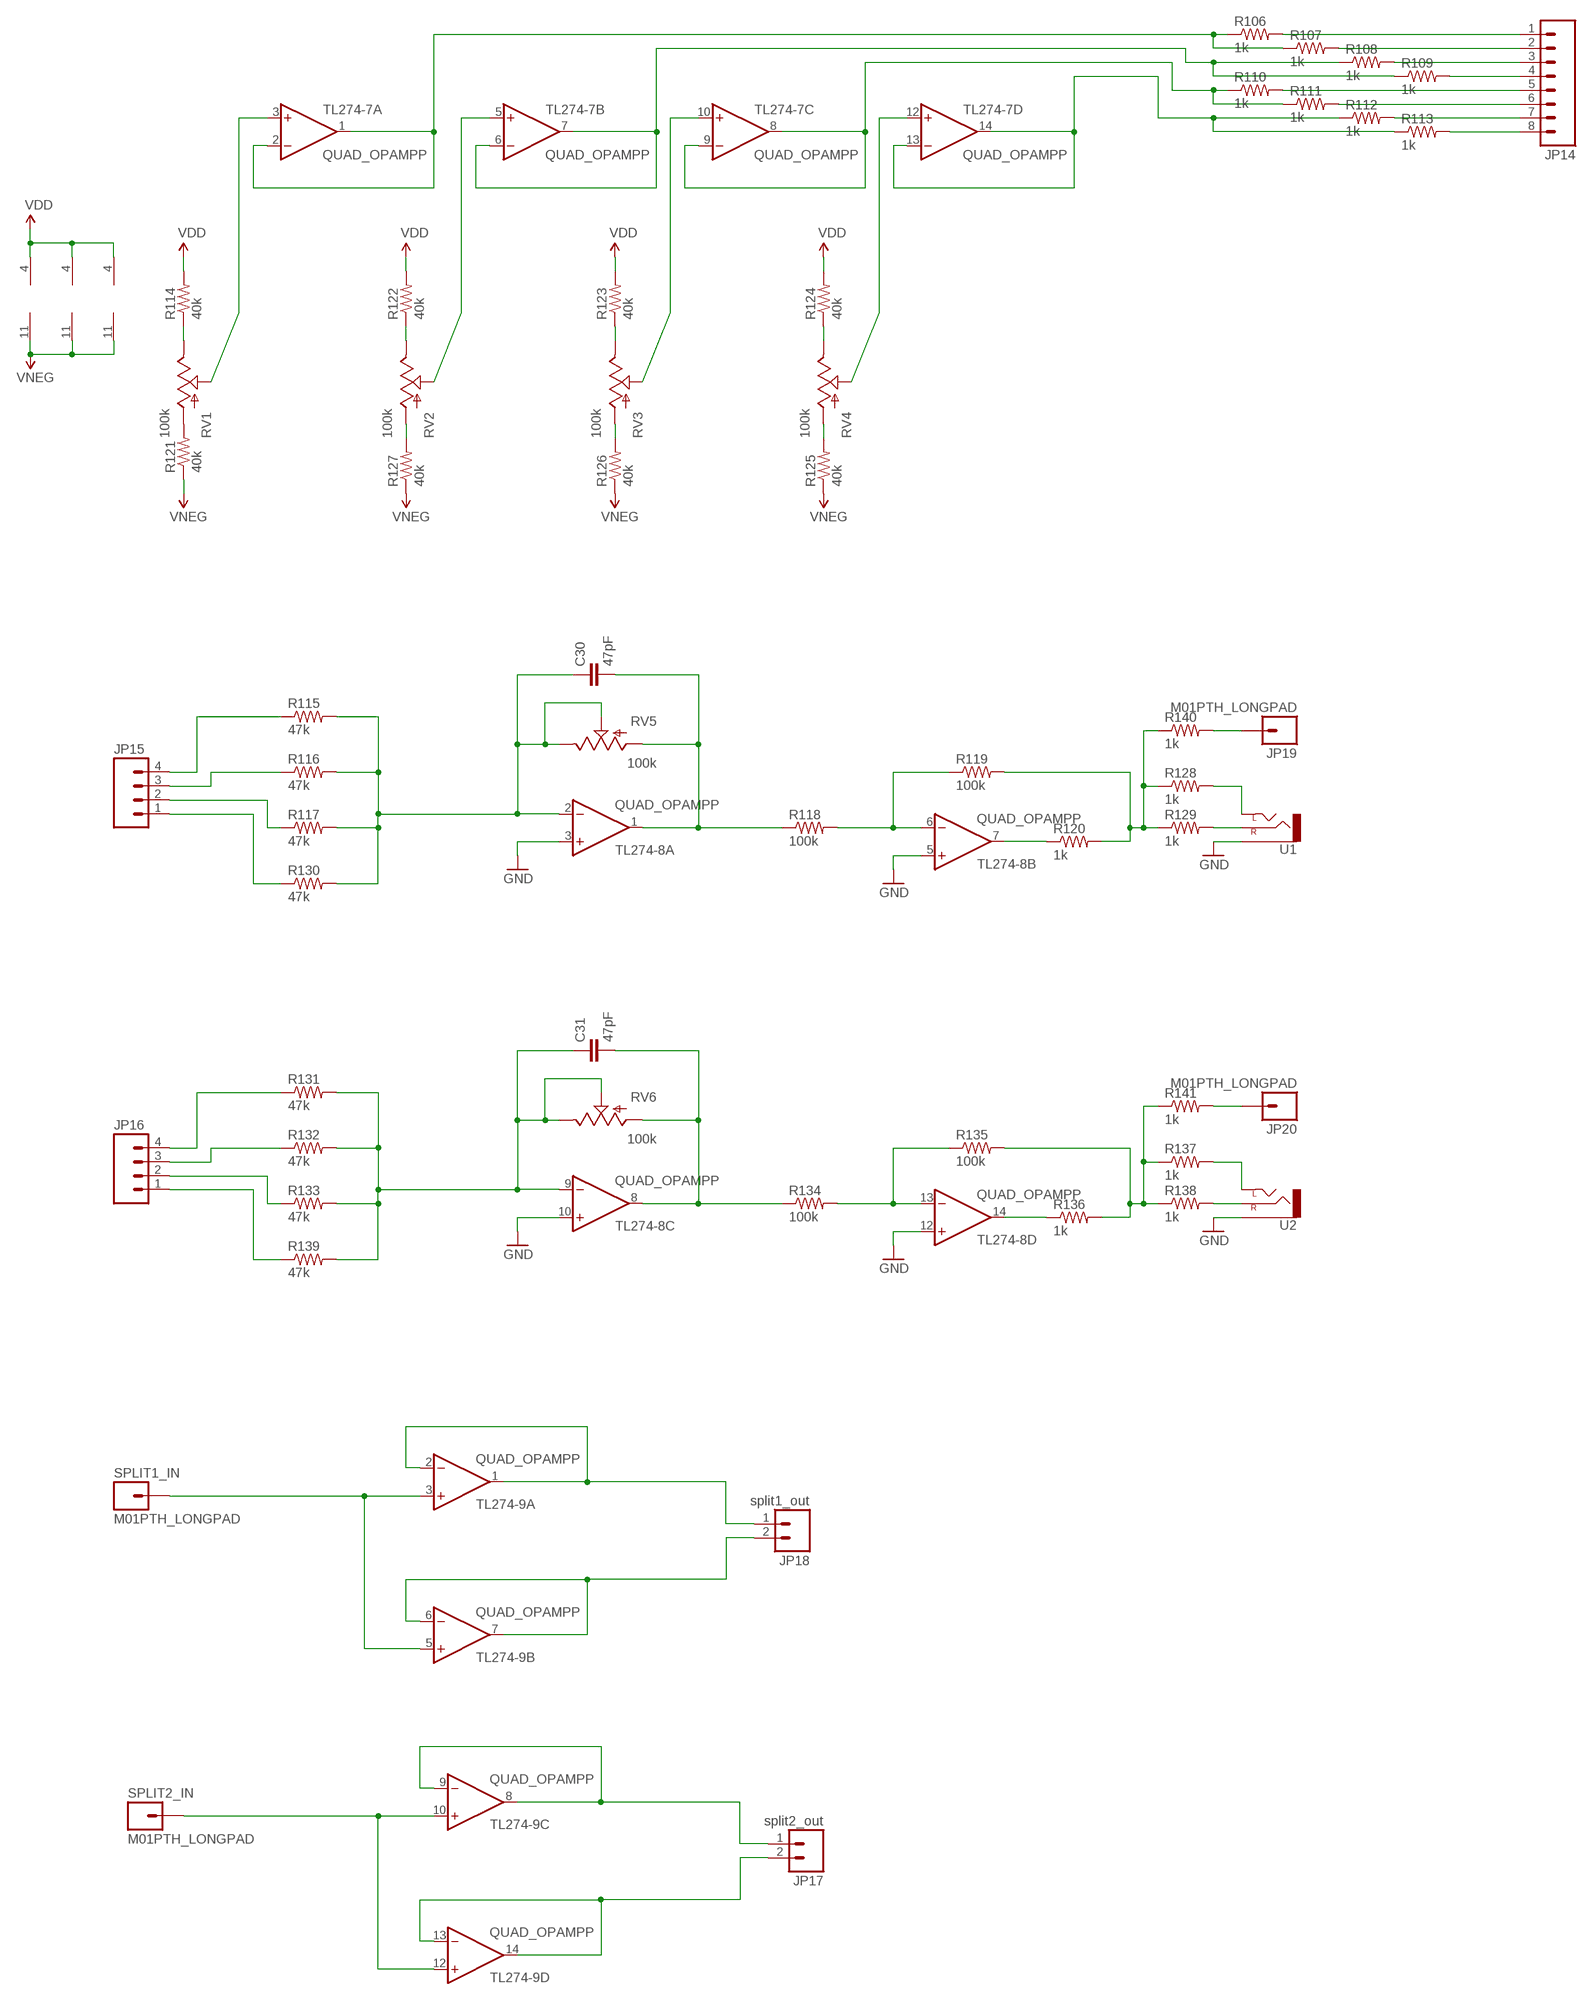
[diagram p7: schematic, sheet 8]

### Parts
C30  47pF  CAPPTH  [CAP-PTH-SMALL]
C31  47pF  CAPPTH  [CAP-PTH-SMALL]
JP14  M08LOCK_LONGPADS  [1X08_LOCK_LONGPADS]
JP15  M04LOCK_LONGPADS  [1X04_LOCK_LONGPADS]
JP16  M04LOCK_LONGPADS  [1X04_LOCK_LONGPADS]
JP17  split2_out  M02LOCK_LONGPADS  [1X02_LOCK_LONGPADS]
JP18  split1_out  M02LOCK_LONGPADS  [1X02_LOCK_LONGPADS]
JP19  M01PTH_LONGPAD  [1X01_LONGPAD]
JP20  M01PTH_LONGPAD  [1X01_LONGPAD]
R106  1k  RESISTORPTH-1/4W  [AXIAL-0.4]
R107  1k  RESISTORPTH-1/4W  [AXIAL-0.4]
R108  1k  RESISTORPTH-1/4W  [AXIAL-0.4]
R109  1k  RESISTORPTH-1/4W  [AXIAL-0.4]
R110  1k  RESISTORPTH-1/4W  [AXIAL-0.4]
R111  1k  RESISTORPTH-1/4W  [AXIAL-0.4]
R112  1k  RESISTORPTH-1/4W  [AXIAL-0.4]
R113  1k  RESISTORPTH-1/4W  [AXIAL-0.4]
R114  40k  RESISTORPTH-1/4W  [AXIAL-0.4]
R115  47k  RESISTORPTH-1/4W  [AXIAL-0.4]
R116  47k  RESISTORPTH-1/4W  [AXIAL-0.4]
R117  47k  RESISTORPTH-1/4W  [AXIAL-0.4]
R118  100k  RESISTORPTH-1/4W  [AXIAL-0.4]
R119  100k  RESISTORPTH-1/4W  [AXIAL-0.4]
R120  1k  RESISTORPTH-1/4W  [AXIAL-0.4]
R121  40k  RESISTORPTH-1/4W  [AXIAL-0.4]
R122  40k  RESISTORPTH-1/4W  [AXIAL-0.4]
R123  40k  RESISTORPTH-1/4W  [AXIAL-0.4]
R124  40k  RESISTORPTH-1/4W  [AXIAL-0.4]
R125  40k  RESISTORPTH-1/4W  [AXIAL-0.4]
R126  40k  RESISTORPTH-1/4W  [AXIAL-0.4]
R127  40k  RESISTORPTH-1/4W  [AXIAL-0.4]
R128  1k  RESISTORPTH-1/4W  [AXIAL-0.4]
R129  1k  RESISTORPTH-1/4W  [AXIAL-0.4]
R130  47k  RESISTORPTH-1/4W  [AXIAL-0.4]
R131  47k  RESISTORPTH-1/4W  [AXIAL-0.4]
R132  47k  RESISTORPTH-1/4W  [AXIAL-0.4]
R133  47k  RESISTORPTH-1/4W  [AXIAL-0.4]
R134  100k  RESISTORPTH-1/4W  [AXIAL-0.4]
R135  100k  RESISTORPTH-1/4W  [AXIAL-0.4]
R136  1k  RESISTORPTH-1/4W  [AXIAL-0.4]
R137  1k  RESISTORPTH-1/4W  [AXIAL-0.4]
R138  1k  RESISTORPTH-1/4W  [AXIAL-0.4]
R139  47k  RESISTORPTH-1/4W  [AXIAL-0.4]
R140  1k  RESISTORPTH-1/4W  [AXIAL-0.4]
R141  1k  RESISTORPTH-1/4W  [AXIAL-0.4]
RV1  100k  POTALPHA_RV09  [ALPS_POT_KIT]
RV2  100k  POTALPS-KIT  [ALPS_POT_KIT]
RV3  100k  POTALPS-KIT  [ALPS_POT_KIT]
RV4  100k  POTALPS-KIT  [ALPS_POT_KIT]
RV5  100k  POTALPS-KIT  [ALPS_POT_KIT]
RV6  100k  POTALPS-KIT  [ALPS_POT_KIT]
SPLIT1_IN  M01PTH_LONGPAD  [1X01_LONGPAD]
SPLIT2_IN  M01PTH_LONGPAD  [1X01_LONGPAD]
TL274-7  QUAD_OPAMPP  [DIL14]
TL274-8  QUAD_OPAMPP  [DIL14]
TL274-9  QUAD_OPAMPP  [DIL14]
U1  AUDIO-JACKPTH  [AUDIO-JACK]
U2  AUDIO-JACKPTH  [AUDIO-JACK]

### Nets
GND: TL274-8.3(A:+IN) TL274-8.5(B:+IN) TL274-8.10(C:+IN) TL274-8.12(D:+IN) U1.SLEEVE U2.SLEEVE ; also sheet 1,2,3,4,5,6,7
N$154: RV1.P$2(S) TL274-7.3(A:+IN)
N$157: R106.P$1 R107.P$1 TL274-7.1(A:OUT) TL274-7.2(A:-IN)
N$158: RV2.P$2(S) TL274-7.5(B:+IN)
N$160: R108.P$1 R109.P$1 TL274-7.6(B:-IN) TL274-7.7(B:OUT)
N$161: RV3.P$2(S) TL274-7.10(C:+IN)
N$162: R110.P$1 R111.P$1 TL274-7.8(C:OUT) TL274-7.9(C:-IN)
N$163: RV4.P$2(S) TL274-7.12(D:+IN)
N$164: R112.P$1 R113.P$1 TL274-7.13(D:-IN) TL274-7.14(D:OUT)
N$165: JP14.1 R106.P$2
N$166: JP14.2 R107.P$2
N$167: JP14.3 R108.P$2
N$168: JP14.4 R109.P$2
N$169: JP14.5 R110.P$2
N$170: JP14.6 R111.P$2
N$171: JP14.7 R112.P$2
N$172: JP14.8 R113.P$2
N$173: C30.1 R115.P$2 R116.P$2 R117.P$2 R130.P$2 RV5.P$1(E) RV5.P$2(S) TL274-8.2(A:-IN)
N$174: C30.2 R118.P$1 RV5.P$3(A) TL274-8.1(A:OUT)
N$175: JP15.4 R115.P$1
N$176: JP15.3 R116.P$1
N$177: JP15.2 R117.P$1
N$178: R118.P$2 R119.P$1 TL274-8.6(B:-IN)
N$179: R119.P$2 R120.P$2 R128.P$1 R129.P$1 R140.P$1
N$180: R120.P$1 TL274-8.7(B:OUT)
N$181: R121.P$2 RV1.P$3(A)
N$182: R114.P$1 RV1.P$1(E)
N$183: R122.P$1 RV2.P$1(E)
N$184: R123.P$1 RV3.P$1(E)
N$185: R124.P$1 RV4.P$1(E)
N$186: R125.P$2 RV4.P$3(A)
N$187: R126.P$2 RV3.P$3(A)
N$188: R127.P$2 RV2.P$3(A)
N$189: R128.P$2 U1.TIP(LEFT)
N$190: R129.P$2 U1.RING(RIGHT)
N$191: JP15.1 R130.P$1
N$192: C31.1 R131.P$2 R132.P$2 R133.P$2 R139.P$2 RV6.P$1(E) RV6.P$2(S) TL274-8.9(C:-IN)
N$193: C31.2 R134.P$1 RV6.P$3(A) TL274-8.8(C:OUT)
N$194: JP16.4 R131.P$1
N$195: JP16.3 R132.P$1
N$196: JP16.2 R133.P$1
N$197: R134.P$2 R135.P$1 TL274-8.13(D:-IN)
N$198: R135.P$2 R136.P$2 R137.P$1 R138.P$1 R141.P$1
N$199: R136.P$1 TL274-8.14(D:OUT)
N$200: R137.P$2 U2.TIP(LEFT)
N$201: R138.P$2 U2.RING(RIGHT)
N$202: JP16.1 R139.P$1
N$203: SPLIT1_IN.1 TL274-9.3(A:+IN) TL274-9.5(B:+IN)
N$204: JP18.1 TL274-9.1(A:OUT) TL274-9.2(A:-IN)
N$205: SPLIT2_IN.1 TL274-9.10(C:+IN) TL274-9.12(D:+IN)
N$206: JP17.1 TL274-9.8(C:OUT) TL274-9.9(C:-IN)
N$207: JP18.2 TL274-9.6(B:-IN) TL274-9.7(B:OUT)
N$208: JP17.2 TL274-9.13(D:-IN) TL274-9.14(D:OUT)
N$209: JP20.1 R141.P$2
N$210: JP19.1 R140.P$2
VDD: R114.P$2 R122.P$2 R123.P$2 R124.P$2 TL274-7.4(P:V+) TL274-8.4(P:V+) TL274-9.4(P:V+) ; also sheet 1,2,3,4,5,6,7
VNEG: R121.P$1 R125.P$1 R126.P$1 R127.P$1 TL274-7.11(P:V-) TL274-8.11(P:V-) TL274-9.11(P:V-) ; also sheet 1,2,3,4,5,6,7

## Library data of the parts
2N3904 2N3904-1-2N3904-5 = SparkFun-DiscreteSemi:TRANSISTOR_NPN: Generic NPN BJT MMBT2222A - TRANS-08049 (SOT-23, 1A 40V) MPSA42 - TRANS-09116 (SOT-23, 500mA 300V) MMBT5088LT1G - TRANS-11160 (SOT-23, 50 mA 30V) BC547 - COM-08928 (TO-92 45V 100mA) (1.Collector 2.Base 3.Emitter) 2N3904 - COM-00521 (TO-92 40V 200mA) (1.Emitter 2.Base 3.Collector) P2N2222A -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
5K 5K1-5K3 10K 10K1 10K-2 500 = SparkFun:TRIMPOT
555 555-1 = SparkFun-AnalogIC:NE555: General purpose bipolar Timer; MF: Arrow Electronics; MPN: NE555N; OC_FARNELL: 1467742; OC_NEWARK: 89K1486
ATT ATT1 ATTACK ATTACK1 CUTOFF DECAY DECAY1 RELEASE RELEASE1 RES0NANCE RV1-RV6 SUSTAIN SUSTAIN1 = SparkFun-Electromechanical:POT
AUDIO_IN AUDIO_OUT JP19 JP20 SPLIT1_IN SPLIT2_IN TRIG_IN TRIG_IN1 = SparkFun:M01: Header 1
C1-C31 = SparkFun:CAP: Capacitor
CA3046 CA3046-2 = synthdiy:CA3046: NPN Transistor Array
CVS CVS1 = SparkFun:M05: Header 5 Standard 5-pin 0.1" header. Use with straight break away headers (SKU : PRT-00116), right angle break away headers (PRT-00553), swiss pins (PRT-00743), machine pins (PRT-00117), and female headers (PRT-00115). Molex polarized connector foot print use with SKU : PRT-08230 with associated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
D1-D17 = SparkFun:DIODE: Diode
DUALOPAMP = SparkFun:OPAMP-DUAL: Operational Amplifier
J1 = SparkFun:POWER_JACK: Power Jack This is the standard 5.5mm barrel jack for power. The PTH is the most common, proven, reliable, footprint. All others are experimental. The Slot footprint only works if the mill layer is transmitted to the PCB fab house so be warned. Spark Fun Electronics SKU : PRT-00119. Mating wall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
J112 Q2 = transistor-fet:?20*: TEMIC / Siliconix N-Channel JFET Source: JFET-J201_Siliconix_data.pdf
JP1 JP3 JP4 JP9 JP10 JP12 JP13 = SparkFun:M03: Header 3 Standard 3-pin 0.1" header. Use with straight break away headers (SKU : PRT-00116), right angle break away headers (PRT-00553), swiss pins (PRT-00743), machine pins (PRT-00117), and female headers (PRT-00115). Molex polarized connector foot print use with SKU : PRT-08232 with associated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
JP2 JP5 JP7 JP8 JP11 JP17 JP18 = SparkFun:M02: Header 2
JP6 = SparkFun-Connectors:M01: Header 1
JP14 = SparkFun:M08: Header 8 Standard 8-pin 0.1" header. Use with straight break away headers (SKU : PRT-00116), right angle break away headers (PRT-00553), swiss pins (PRT-00743), machine pins (PRT-00117), and female headers (PRT-00115).
JP15 JP16 = SparkFun:M04: Header 4 Standard 4-pin 0.1" header. Use with straight break away headers (SKU : PRT-00116), right angle break away headers (PRT-00553), swiss pins (PRT-00743), machine pins (PRT-00117), and female headers (PRT-00115). Molex polarized connector foot print use with SKU : PRT-08231 with associated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
LED1 = adafruit:LED: LED
LM7809 LM7909 = SparkFun:V_REG_78XX: Voltage Regulator Standard 7805 5V regulator. IGO (Input Ground Output). Spark Fun Electronics SKU : COM-00107
LM13700 = synthdiy:LM13700: National Dual OTA with buffers.
R1-R141 = SparkFun:RESISTOR: Resistor
S1 S2 = SparkFun-Electromechanical:SWITCH-MOMENTARY-2: Various NO switches- pushbuttons, reed, etc; PROD_ID: SWCH-09185
THAT2180 = resistor-sil:E4R: SIL RESISTOR; OC_FARNELL: unknown; OC_NEWARK: unknown
TL274 TL274-1-TL274-9 = adafruit:QUAD_OPAMP: OP AMP Standard quad package
U1 U2 = SparkFun:AUDIO-JACK: 3.5mm Audio Jack Simple 3.5mm common PCB mount audio jack. SKU: PRT-08032

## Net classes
0 default: width 0.356 mm, clearance 0.254 mm

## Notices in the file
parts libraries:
SparkFun: Licensing: CC v3.0 Share-Alike You are welcome to use this library for commercial purposes.
SparkFun-Aesthetics: Licensing: Creative Commons ShareAlike 4.0 International - https://creativecommons.org/licenses/by-sa/4.0
